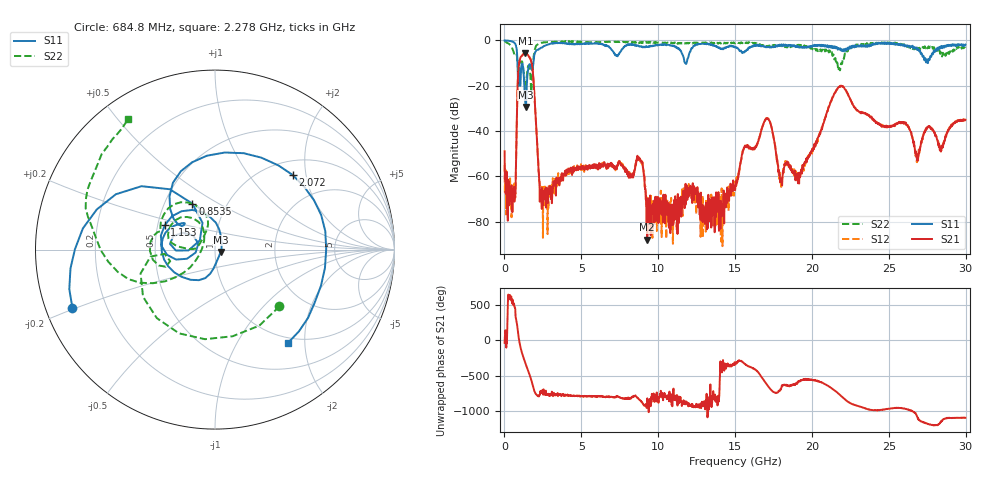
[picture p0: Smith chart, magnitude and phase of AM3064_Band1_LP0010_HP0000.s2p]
# Hz S DB R 50.0
!freq dBS11 angS11 dBS21 angS21 dBS12 angS12 dBS22 angS22
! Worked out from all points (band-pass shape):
!   1600 points, 10 MHz to 29.98 GHz, reference 50 ohm
!   highest |S21| = -5.57 dB at 1.36 GHz (marker M1); lowest = -87.9 dB at 9.288 GHz (marker M2)
!   |S21| within 3 dB of the highest: 998.1 MHz to 1.711 GHz (713.3 MHz wide, 52.7 % of centre)
!   lowest |S11| = -29.4 dB at 1.397 GHz (marker M3), VSWR 1.07, Z = 53.2 - j1.41 ohm
!   |S11| at or under -10 dB: 848.5 MHz to 1.877 GHz (1.028 GHz wide, 75.5 % of centre); 11.75 GHz to 11.84 GHz (91.97 MHz wide, 0.78 % of centre); 27.54271 GHz to 27.54472 GHz (2.007 MHz wide, 0.00729 % of centre)
!   |S22| runs from -22.8 to -0.3 dB; largest |S21 - S12| = 0.0065
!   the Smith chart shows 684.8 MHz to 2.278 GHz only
!   S11 on the Smith chart (normalised r, x): 684.8 MHz: 0.08, -0.20; 853.5 MHz: 0.69, +0.38; 1.153 GHz: 0.55, +0.17; 2.072 GHz: 1.29, +1.68; 2.278 GHz: 0.91, -1.67
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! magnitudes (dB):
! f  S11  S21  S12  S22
! 10 MHz  0.0  -48.9  -54.9  -0.3
! 328.6 MHz  -0.2  -66.6  -64.5  -1.7
! 684.8 MHz  -1.3  -66.9  -67.0  -6.4
! 853.5 MHz  -10.9  -20.4  -20.3  -11.0
! 1.153 GHz  -10.1  -6.7  -6.6  -9.4
! 1.36 GHz  -27.5  -5.6  -5.6  -20.9
! 1.397 GHz  -29.4  -5.6  -5.6  -19.3
! 1.772 GHz  -12.9  -10.1  -10.1  -20.4
! 2.072 GHz  -4.4  -39.1  -38.8  -2.2
! 2.278 GHz  -3.6  -62.2  -62.6  -1.2
! 5.015 GHz  -1.5  -56.4  -55.3  -0.6
! 8.782 GHz  -2.7  -51.8  -52.8  -0.8
! 9.288 GHz  -2.9  -87.9  -84.7  -1.0
! 10 GHz  -2.0  -69.1  -77.6  -0.9
! 15 GHz  -2.9  -66.0  -62.2  -1.3
! 17.05 GHz  -2.9  -34.5  -34.4  -2.7
! 17.97 GHz  -2.4  -61.6  -62.7  -2.1
! 19.99 GHz  -2.8  -48.5  -49.0  -3.4
! 21.85 GHz  -3.5  -20.2  -20.0  -12.5
! 25 GHz  -1.0  -38.0  -38.0  -1.2
! 26.87 GHz  -4.1  -53.1  -53.8  -3.2
! 29.98 GHz  -1.8  -35.0  -35.3  -3.2
